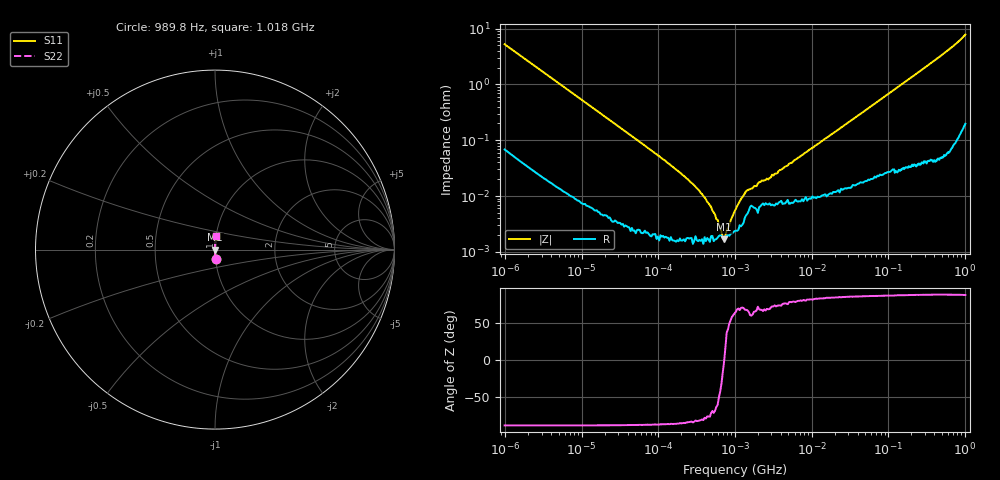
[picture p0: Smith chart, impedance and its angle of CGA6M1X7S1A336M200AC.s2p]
! S-Parameter Data Generated by TDK Corporation
! Copyright(C) 2024 TDK Corporation.
! All Rights Reserved.
! TDK P/N: CGA6M1X7S1A336M200AC (Multilayer Ceramic Chip Capacitor)
! Property: C=33uF
! Size(LxWxT): 3.2x2.5x2mm
! Model Type: s2p (Touchstone File Format Version 1.0)
! Frequency: DC=Yes Start=0.000989846MHz Stop=1017.91MHz 409points Log-sweep
! Model Generated on May 28, 2024
! Terms and conditions regarding TDK Simulation Models:
! 1)This simulation model is being provided solely for informational
!  purposes. Please refer to the specifications of the products in
!  terms of detailed characteristics of such products.
! 2)In no event shall TDK Corporation of any of its subsidiaries be
!  liable for any loss or damage arising, directly or indirectly,
!  from any information contained in this simulation model, including,
!  but not limited to loss or damages arising from any inaccuracies,
!  omissions or errors in connection with such information.
! 3)Any and all copyrights on this simulation model are owned by
!  TDK Corporation.  Duplication or redistribution of this simulation
!  model without prior written permission from TDK Corporation
!  is prohibited.
! 4)This simulation model is subject to any modification or change
!  without any prior notice.
! 5)Neither TDK Corporation nor any of its subsidiaries shall make any
!  warranty, express or implied, including but not limited to the
!  correctness, implied warranties of merchantability and fitness for
!  a particular purpose with respect to this simulation models.
! 6)The use of this simulation model shall be deemed to have consented
!  to the terms and conditions hereof.
! Port Assignments:
!  1 ---| |--- 2
! Applicable Conditions:
!  Temperature = 25 degC
!  DC Bias Voltage = 0 V
!  Small Signal Operation
# Hz S MA R 50
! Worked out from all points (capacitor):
!   408 points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, 989.8 Hz to 1.018 GHz, reference 50 ohm
!   read as one part in series: C = 30.6 uF near 1.07 kHz
!   lowest |Z| = 1.68 mohm at 723.3 kHz (marker M1)
!   series resonance near 726 kHz, so ESL is about 1.6 nH
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989.846  0.05222 -86.3  0.998 3.0  0.998 3.0  0.05222 -86.3
1070.18  0.04837 -86.5  0.9982 2.8  0.9982 2.8  0.04837 -86.5
2625.44  0.01996 -88.1  0.9995 1.1  0.9995 1.1  0.01996 -88.1
10287  0.005158 -88.9  0.9999 0.3  0.9999 0.3  0.005158 -88.9
102818  0.0005179 -88.2  1 0.0  1 0.0  0.0005179 -88.2
233303  0.0002076 -85.2  1 0.0  1 0.0  0.0002076 -85.2
294844  0.0001547 -84.1  1 0.0  1 0.0  0.0001547 -84.1
387446  9.984e-05 -82.0  1 0.0  1 0.0  9.984e-05 -82.0
418891  8.797e-05 -79.8  1 0.0  1 0.0  8.797e-05 -79.8
723330  1.683e-05 -2.0  1 0.0  1 0.0  1.683e-05 -2.0
1027650  5.817e-05 65.7  1 -0.0  1 -0.0  5.817e-05 65.7
1249030  9.554e-05 71.4  1 -0.0  1 -0.0  9.554e-05 71.4
1518090  0.0001307 65.5  0.9999 -0.0  0.9999 -0.0  0.0001307 65.5
1774520  0.00015 65.7  0.9999 -0.0  0.9999 -0.0  0.00015 65.7
2156790  0.0001787 68.5  0.9999 -0.0  0.9999 -0.0  0.0001787 68.5
2725710  0.0001985 69.2  0.9999 -0.0  0.9999 -0.0  0.0001985 69.2
2946930  0.0002162 71.6  0.9999 -0.0  0.9999 -0.0  0.0002162 71.6
1.02712e7  0.0007309 82.2  0.9999 -0.0  0.9999 -0.0  0.0007309 82.2
1.0266e8  0.006852 87.4  0.9997 -0.4  0.9997 -0.4  0.006852 87.4
5.25832e8  0.03526 87.2  0.9989 -2.0  0.9989 -2.0  0.03526 87.2
7.69149e8  0.05349 85.9  0.9976 -3.1  0.9976 -3.1  0.05349 85.9
1.01791e9  0.07797 84.1  0.995 -4.5  0.995 -4.5  0.07797 84.1
